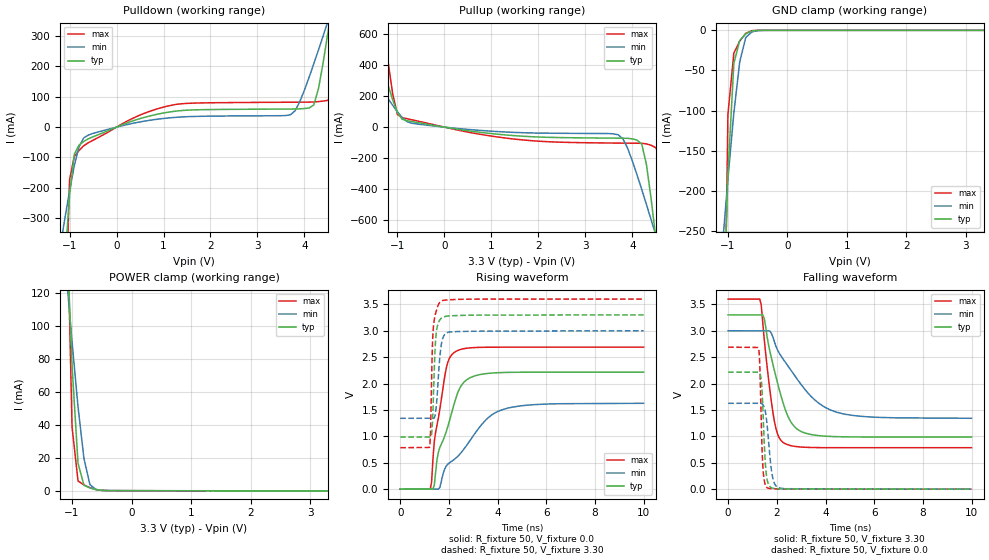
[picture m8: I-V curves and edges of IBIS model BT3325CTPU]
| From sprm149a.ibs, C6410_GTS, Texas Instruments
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[Model]   BT3325CTPU
Model_type   I/O
Vinh = 2.00
Vinl = 0.80
Enable   Active-Low
Polarity   Non-Inverting
| signals   A, GZ, Y
Vmeas = 1.5
|   typ   min   max
C_comp   1.6130p   1.5354p   1.7989p
|   typ   min   max
[Temperature Range]   25   -40   125
|   typ   min   max
[Voltage Range]   3.30V   3.00V   3.60V
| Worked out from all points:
|   slope of the pulldown table from 0 to 0.495 V, typ, clamps not added: 17.7 ohm
|   slope of the pullup table from 0 to 0.495 V, typ, clamps not added: 21.6 ohm
|   GND clamp passes 1 mA (typ) near -0.60 V on its own axis
|   POWER clamp passes 1 mA (typ) near -0.63 V on its own axis
|   rising waveform, R_fixture 50, V_fixture 0.0: 20-80 % time 840ps typ, 1.71ns min, 495ps max; typ from 0 V to 2.22 V
|   falling waveform, R_fixture 50, V_fixture 3.30: 20-80 % time 775ps typ, 1.6ns min, 432ps max; typ from 3.3 V to 0.987 V
|   rising waveform, R_fixture 50, V_fixture 3.30: 20-80 % time 116ps typ, 165ps min, 101ps max; typ from 0.987 V to 3.3 V
|   falling waveform, R_fixture 50, V_fixture 0.0: 20-80 % time 132ps typ, 209ps min, 100ps max; typ from 2.22 V to 0 V
[Pulldown]
|   Voltage   I(typ)   I(min)   I(max)
-3.3V     -6.78A     -2.576A    -22.51A
-1.1V     -449.6mA   -301.3mA   -716.1mA
-900mV    -90.04mA   -128.4mA   -97.36mA
-600mV    -38.44mA   -26.14mA   -51.28mA
1.2V      51.55mA    31.56mA    73.11mA
3.7V      59.71mA    40.53mA    82.18mA
4.2V      73.24mA    209.3mA    83.11mA
4.5V      311.9mA    348.7mA    88.35mA
4.6V      415.1mA    396.2mA    114.8mA
4.7V      521.2mA    444mA      265.5mA
4.8V      629mA      492mA      482.1mA
6.6V      2.641A     1.373A     5.229A
[GND_clamp]
|   Voltage   I(typ)   I(min)   I(max)
-3.3V     -6.723A    -2.538A    -22.45A
-1.1V     -408.3mA   -276.5mA   -658.1mA
-1V       -181mA     -185.7mA   -105.4mA
-900mV    -41.22mA   -103.1mA   -28.36mA
-800mV    -12.49mA   -38.76mA   -13.32mA
-700mV    -4.472mA   -9.073mA   -3.784mA
-600mV    -854.1uA   -2.124mA   -419.5uA
-400mV    -4.328uA   -46.41uA   -434.3nA
3.3V      88.82pA    2.083uA    133.2pA
[Pullup]
|   Voltage   I(typ)   I(min)   I(max)
-3.3V     2.595A     1.198A     5.975A
-2.2V     1.359A     659.7mA    3.015A
-1.6V     695.4mA    370.8mA    1.426A
-1.3V     373.9mA    230.2mA    662.2mA
-1V       93.9mA     99.07mA    81.14mA
-800mV    41.97mA    36.23mA    54.79mA
3.7V      -71.34mA   -49.45mA   -103.2mA
4.1V      -83.89mA   -308.7mA   -104.2mA
4.5V      -720.2mA   -699.7mA   -132.7mA
4.6V      -989mA     -800.8mA   -203.6mA
4.7V      -1.265A    -902.5mA   -740.4mA
6.6V      -6.776A    -2.885A    -19.48A
[POWER_clamp]
|   Voltage   I(typ)   I(min)   I(max)
-3.3V     2.59A      1.192A     5.973A
-1.1V     164.2mA    133.3mA    197.3mA
-1V       76.2mA     90.47mA    38.64mA
-900mV    16.71mA    51.17mA    5.958mA
-800mV    3.31mA     19.53mA    3.455mA
-700mV    1.625mA    3.736mA    1.82mA
-600mV    707.1uA    738uA      679.1uA
-500mV    198.8uA    185uA      148.9uA
3.3V      -108.4uA   -67.78uA   -162.2uA
[Ramp]
|   I(typ)   I(min)   I(max)
dV/dt_r   1.330/0.841n   0.976/1.713n   1.614/0.495n
dV/dt_f   1.388/0.776n   0.995/1.604n   1.689/0.432n
[Rising Waveform]
R_fixture = 50
V_fixture = 0.0
|  pu_on
|  TIME   V(typ)   V(min)   V(max)
0s        2nV        12nV       1nV
1.233ns   2.493mV    1.669mV    1.411nV
1.289ns   2.493mV    1.848mV    132.6mV
1.4ns     79.52mV    1.848mV    905.2mV
1.566ns   698.4mV    1.848mV    1.348V
1.844ns   1.028V     399.8mV    2.181V
2.289ns   1.727V     589.8mV    2.61V
2.845ns   2.104V     906.8mV    2.675V
4.234ns   2.209V     1.511V     2.689V
10ns      2.216V     1.626V     2.689V
[Falling Waveform]
R_fixture = 50
V_fixture = 3.30
V_fixture_min = 3.00
V_fixture_max = 3.60
|  pd_on
|  TIME   V(typ)   V(min)   V(max)
0s        3.3V       3V         3.6V
1.298ns   3.3V       2.998V     3.6V
1.359ns   3.3V       2.998V     3.489V
1.48ns    3.238V     2.998V     2.851V
1.842ns   2.358V     2.876V     1.443V
2.023ns   2.022V     2.641V     1.054V
2.265ns   1.622V     2.459V     882.5mV
2.869ns   1.126V     2.062V     802.7mV
4.44ns    994.6mV    1.46V      785.5mV
10ns      986.8mV    1.342V     785.2mV
[Rising Waveform]
R_fixture = 50
V_fixture = 3.30
V_fixture_min = 3.00
V_fixture_max = 3.60
|  pd_off
|  TIME   V(typ)   V(min)   V(max)
0s        986.8mV    1.342V     785.2mV
1.2ns     986.8mV    1.343V     790.5mV
1.242ns   986.8mV    1.343V     1.066V
1.304ns   1.113V     1.343V     2.422V
1.367ns   1.828V     1.343V     3.098V
1.43ns    2.636V     1.395V     3.283V
1.471ns   2.923V     1.528V     3.361V
1.68ns    3.234V     2.716V     3.561V
2.056ns   3.282V     2.978V     3.587V
10ns      3.3V       3V         3.6V
[Falling Waveform]
R_fixture = 50
V_fixture = 0.0
|  pu_off
|  TIME   V(typ)   V(min)   V(max)
0s        2.216V     1.626V     2.689V
1.25ns    2.216V     1.626V     2.657V
1.298ns   2.19V      1.626V     2.364V
1.371ns   2.019V     1.624V     1.095V
1.431ns   1.469V     1.595V     388.2mV
1.528ns   486mV      1.468V     82.34mV
1.612ns   157.1mV    1.157V     25.33mV
1.818ns   20.68mV    245.2mV    8.16mV
2.108ns   6.986mV    23.8mV     4.329mV
10ns      472.4nV    5.476uV    257.5nV
